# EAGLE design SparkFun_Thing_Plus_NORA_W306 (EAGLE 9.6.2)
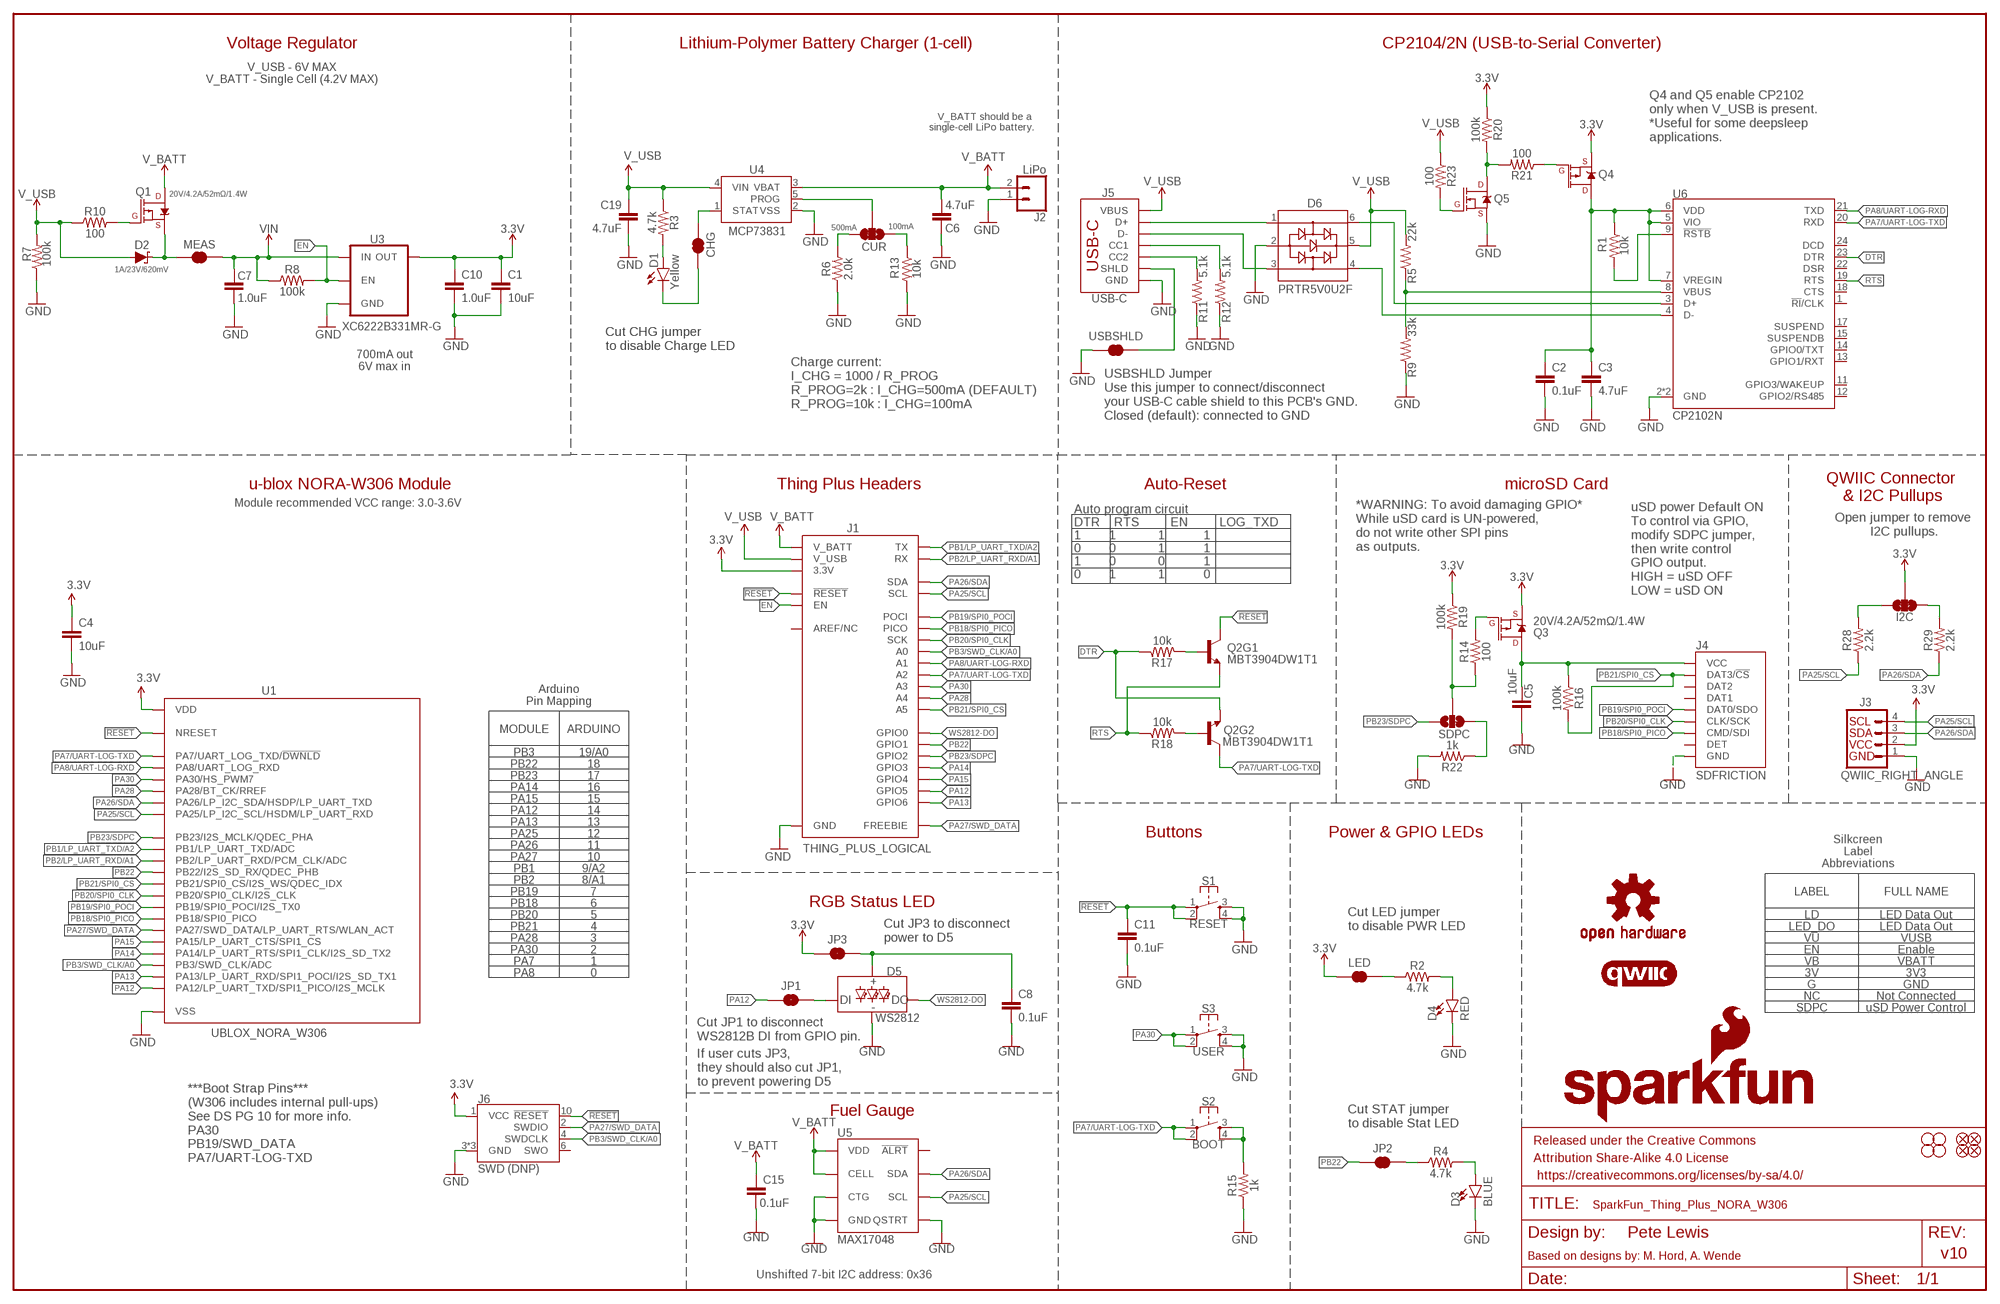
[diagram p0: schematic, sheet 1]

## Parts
C1  10uF  10UF-0402T-6.3V-20%  [0402-TIGHT]
C2  0.1uF  0.1UF-0402T-16V-10%  [0402-TIGHT]
C3  4.7uF  4.7UF-0603-35V-(20%)  [0603]
C4  10uF  10UF-0402T-6.3V-20%  [0402-TIGHT]
C5  10uF  10UF-0402T-6.3V-20%  [0402-TIGHT]
C6  4.7uF  4.7UF-0603-35V-(20%)  [0603]
C7  1.0uF  1.0UF-0402T-16V-10%  [0402-TIGHT]
C8  0.1uF  0.1UF-0402T-16V-10%  [0402-TIGHT]
C10  1.0uF  1.0UF-0402T-16V-10%  [0402-TIGHT]
C11  0.1uF  0.1UF-0402T-16V-10%  [0402-TIGHT]
C15  0.1uF  0.1UF-0402T-16V-10%  [0402-TIGHT]
C19  4.7uF  4.7UF-0603-35V-(20%)  [0603]
CHG  JUMPER-SMT_2_NC_TRACE_SILK  [SMT-JUMPER_2_NC_TRACE_SILK]
CUR  JUMPER-SMT_3_1-NC_TRACE_SILK  [SMT-JUMPER_3_1-NC_TRACE_SILK]
D1  Yellow  LED-YELLOW0603  [LED-0603]
D2  1A/23V/620mV  DIODE-SCHOTTKY-BAT20J  [SOD-323]
D3  BLUE  LED-BLUE0603  [LED-0603]
D4  RED  LED-RED_0603-KB  [LED-0603]
D5  WS2812  WS2812_2020  [WS2812-2020]
D6  PRTR5V0U2F  [SOT886]
FD1  FIDUCIALUFIDUCIAL  [FIDUCIAL-MICRO]
FD2  FIDUCIALUFIDUCIAL  [FIDUCIAL-MICRO]
FD3  FIDUCIALUFIDUCIAL  [FIDUCIAL-MICRO]
FD4  FIDUCIALUFIDUCIAL  [FIDUCIAL-MICRO]
FRAME1  FRAME-LEDGER  [CREATIVE_COMMONS]
H1  STAND-OFF  [STAND-OFF]
H2  STAND-OFF  [STAND-OFF]
H3  STAND-OFF  [STAND-OFF]
H4  STAND-OFF  [STAND-OFF]
I2C  JUMPER-SMT_3_2-NC_TRACE_SILK  [SMT-JUMPER_3_2-NC_TRACE_SILK]
J1  THING_PLUS_LOGICAL  [THING_PLUS]
J2  LiPo  CONN_02-JST-2MM-SMT  [JST-2-SMD]
J3  QWIIC_RIGHT_ANGLE  QWIIC_CONNECTORJS-1MM  [JST04_1MM_RA]
J4  SDFRICTION  MICRO-SDFRICTION  [MICROSD_TINY]
J5  USB-C  USB_C_4-LAYER-ISOLATED  [USB-C-16P-4LAYER-ISOLATED]
J6  SWD (DNP)  CORTEX_JTAG_DEBUG_MINIMUM_SMD_UNSHROUDED_DNP_NO_PASTE  [2X5-SMD-UNSHROUDED_DNP_NO_PASTE]
JP1  JUMPER-SMT_2_NC_TRACE_SILK  [SMT-JUMPER_2_NC_TRACE_SILK]
JP2  JUMPER-SMT_2_NC_TRACE_SILK  [SMT-JUMPER_2_NC_TRACE_SILK]
JP3  JUMPER-SMT_2_NC_TRACE_SILK  [SMT-JUMPER_2_NC_TRACE_SILK]
LED  JUMPER-SMT_2_NC_TRACE_SILK  [SMT-JUMPER_2_NC_TRACE_SILK]
LOGO2  OSHW-LOGOM  [OSHW-LOGO-M]
LOGO3  SFE_LOGO_NAME_FLAME.1_INCH  [SFE_LOGO_NAME_FLAME_.1]
LOGO6  QWIIC_LOGO_4MM  [QWIIC_4MM]
MEAS  JUMPER-COMBO_2_NC_TRACE  [COMBO-JUMPER_2_NC_TRACE]
Q1  20V/4.2A/52mΩ/1.4W  MOSFET_PCH-DMG2305UX-7  [SOT23-3]
Q2  MBT3904DW1T1  TRANS_NPN_DUAL-MBT3904DW1T1  [SC70-6]
Q3  20V/4.2A/52mΩ/1.4W  MOSFET_PCH-DMG2305UX-7  [SOT23-3]
Q4  20V/4.2A/52mΩ/1.4W  MOSFET_PCH-DMG2305UX-7  [SOT23-3]
Q5  20V/0.2A/8MHz/1.2Ω/1Vth  MOSFET-NCH-RE1C002UNTCL  [SOT-416FL]
R1  10k  10KOHM-0402T-1/16W-1%  [0402-TIGHT]
R2  4.7k  4.7KOHM-0402T-1/16W-1%  [0402-TIGHT]
R3  4.7k  4.7KOHM-0402T-1/16W-1%  [0402-TIGHT]
R4  4.7k  4.7KOHM-0402T-1/16W-1%  [0402-TIGHT]
R5  22k  22KOHM-0402_TIGHT-1/10W-1%  [0402-TIGHT]
R6  2.0k  2.0KOHM-0603-1/10W-5%  [0603]
R7  100k  100KOHM-0402T-1/16W-1%  [0402-TIGHT]
R8  100k  100KOHM-0402T-1/16W-1%  [0402-TIGHT]
R9  33k  33KOHM-0402T-1/16W-1%  [0402-TIGHT]
R10  100  100OHM-0402-TIGHT-1/16W-1%  [0402-TIGHT]
R11  5.1k  5.1KOHM-0402T-1/16W-1%  [0402-TIGHT]
R12  5.1k  5.1KOHM-0402T-1/16W-1%  [0402-TIGHT]
R13  10k  10KOHM-0402T-1/16W-1%  [0402-TIGHT]
R14  100  100OHM-0402-TIGHT-1/16W-1%  [0402-TIGHT]
R15  1k  1KOHM-0402T-1/16W-1%  [0402-TIGHT]
R16  100k  100KOHM-0402T-1/16W-1%  [0402-TIGHT]
R17  10k  10KOHM-0402T-1/16W-1%  [0402-TIGHT]
R18  10k  10KOHM-0402T-1/16W-1%  [0402-TIGHT]
R19  100k  100KOHM-0402T-1/16W-1%  [0402-TIGHT]
R20  100k  100KOHM-0402T-1/16W-1%  [0402-TIGHT]
R21  100  100OHM-0402-TIGHT-1/16W-1%  [0402-TIGHT]
R22  1k  1KOHM-0402T-1/16W-1%  [0402-TIGHT]
R23  100  100OHM-0402-TIGHT-1/16W-1%  [0402-TIGHT]
R28  2.2k  2.2KOHM-0402T-1/16W-1%  [0402-TIGHT]
R29  2.2k  2.2KOHM-0402T-1/16W-1%  [0402-TIGHT]
S1  RESET  MOMENTARY-SWITCH-SPST-2-SMD-4.6X2.8MM  [TACTILE_SWITCH_SMD_4.6X2.8MM]
S2  BOOT  MOMENTARY-SWITCH-SPST-2-SMD-4.6X2.8MM  [TACTILE_SWITCH_SMD_4.6X2.8MM]
S3  USER  MOMENTARY-SWITCH-SPST-2-SMD-4.6X2.8MM  [TACTILE_SWITCH_SMD_4.6X2.8MM]
SDPC  JUMPER-SMT_3_1-NC_TRACE_SILK  [SMT-JUMPER_3_1-NC_TRACE_SILK]
U1  UBLOX_NORA_W306  [UBLOX-NORA-W3]
U3  XC6222B331MR-G  [SOT23-5]
U4  MCP73831  [SOT23-5]
U5  MAX17048  MAX17048DFN8  [DFN-8]
U6  CP2102N  [QFN24]
USBSHLD  JUMPER-SMT_2_NC_TRACE_SILK  [SMT-JUMPER_2_NC_TRACE_SILK]

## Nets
3.3V: C1.1 C4.1 C10.1 I2C.2 J1.27(3.3V) J3.2 J6.1(VCC) JP3.1 LED.1 Q3.2(S) Q4.2(S) R19.1 R20.1 U1.A7(VDD) U1.A8(VDD) U1.B7(VDD) U3.5(OUT)
!RESET!: C11.1 J1.28(!RESET) J6.10(!RESET) Q2.3(C) S1.1 S1.2 U1.J3(NRESET)
CC1: J5.A5(CC1) R12.2
CC2: J5.B5(CC2) R11.2
CHG: CHG.2 U4.1(STAT)
DTR: Q2.1(E) R17.1 U6.23(DTR)
EN: J1.11(EN) R8.2 U3.3(EN)
GND: C1.2 C2.2 C3.2 C4.2 C5.2 C6.2 C7.2 C8.2 C10.2 C11.2 C15.2 C19.2 D3.C D4.C D5.GND D6.2 J1.25(GND) J2.1 J3.1 J4.6(GND) J4.GND1(GND) J4.GND2(GND) J4.GND3(GND) J4.GND4(GND) J4.GND5(GND) J4.GND6(GND) J5.GND J5.GND2(GND) J6.3(GND) J6.5(GND) J6.9(GND) Q5.2(S) R6.1 R7.1 R9.1 R11.1 R12.1 R13.2 R15.1 R22.2 S1.3 S1.4 S3.3 S3.4 U1.A1(VSS) U1.A9(VSS) U1.B2(VSS) U1.B8(VSS) U1.E4(VSS) U1.E5(VSS) U1.F4(VSS) U1.F5(VSS) U1.K2(VSS) U1.K3(VSS) U1.K5(VSS) U1.K7(VSS) U1.K8(VSS) U1.L1(VSS) U1.L9(VSS) U1.M1(VSS) U1.M2(VSS) U1.M8(VSS) U1.M9(VSS) U3.2(GND) U4.2(VSS) U5.1(CTG) U5.4(GND) U5.6(QSTRT) U5.9(GND) U6.2(GND) U6.PAD(GND) USBSHLD.1
N$1: R1.2 U6.9(!RSTB)
N$2: D3.A R4.2
N$3: Q2.5(B) R17.2
N$4: R5.1 R9.2 U6.8(VBUS)
N$5: Q2.2(B) R18.2
N$6: CHG.1 D1.C
N$7: Q1.1(G) R10.2
N$8: R15.2 S2.3 S2.4
N$9: CUR.2 U4.5(PROG)
N$10: D5.DI JP1.2
N$11: CUR.1 R13.1
N$12: LED.2 R2.1
N$13: CUR.3 R6.2
N$14: D4.A R2.2
N$15: D6.6 U6.3(D+)
N$16: D6.1 J5.A6(D+) J5.B6(D+)
N$17: D1.A R3.2
N$18: D6.4 U6.4(D-)
N$19: D6.3 J5.A7(D-) J5.B7(D-)
N$20: I2C.3 R28.2
N$21: I2C.1 R29.2
N$22: JP2.2 R4.1
N$23: D2.C MEAS.1 MEAS.3 Q1.2(S)
N$24: Q3.1(G) R14.2
N$25: C5.1 J4.4(VCC) Q3.3(D) R16.1
N$26: R14.1 R19.2 SDPC.2
N$27: Q5.3(D) R20.2 R21.2
N$28: C8.1 D5.VCC JP3.2
N$29: C2.1 C3.1 Q4.3(D) R1.1 U6.5(VIO) U6.6(VDD) U6.7(VREGIN)
N$30: Q4.1(G) R21.1
N$31: Q5.1(G) R23.2
N$32: R22.1 SDPC.3
PA7/UART-LOG-TXD: J1.22(A2) Q2.6(C) S2.1 S2.2 U1.A5(PA7/UART_LOG_TXD/!DWNLD!) U6.20(RXD)
PA8/UART-LOG-RXD: J1.23(A1) U1.A6(PA8/UART_LOG_RXD) U6.21(TXD)
PA12: J1.4(GPIO5) JP1.1 U1.J9(PA12/LP_UART_TXD/SPI1_PICO/I2S_MCLK)
PA13: J1.3(GPIO6) U1.J8(PA13/LP_UART_RXD/SPI1_POCI/I2S_SD_TX1)
PA14: J1.6(GPIO3) U1.H9(PA14/LP_UART_RTS/SPI1_CLK/I2S_SD_TX2)
PA15: J1.5(GPIO4) U1.H8(PA15/LP_UART_CTS/SPI1_CS)
PA25/SCL: J1.2(SCL) J3.4 R28.1 U1.C2(PA25/LP_I2C_SCL/HSDM/LP_UART_RXD) U5.7(SCL)
PA26/SDA: J1.1(SDA) J3.3 R29.1 U1.C1(PA26/LP_I2C_SDA/HSDP/LP_UART_TXD) U5.8(SDA)
PA27/SWD_DATA: J1.13(FREEBIE) J6.2(SWDIO) U1.H2(PA27/SWD_DATA/LP_UART_RTS/WLAN_ACT)
PA28: J1.20(A4) U1.B3(PA28/BT_CK/RREF)
PA30: J1.21(A3) S3.1 S3.2 U1.B1(PA30/HS_PWM7)
PB1/LP_UART_TXD/A2: J1.14(TX) U1.D8(PB1/LP_UART_TXD/ADC)
PB2/LP_UART_RXD/A1: J1.15(RX) U1.E8(PB2/LP_UART_RXD/PCM_CLK/ADC)
PB3/SWD_CLK/A0: J1.24(A0) J6.4(SWDCLK) U1.J2(PB3/SWD_CLK/ADC)
PB18/SPI0_PICO: J1.17(PICO) J4.3(CMD/SDI) U1.G9(PB18/SPI0_PICO)
PB19/SPI0_POCI: J1.16(POCI) J4.7(DAT0/SDO) U1.G8(PB19/SPI0_POCI/I2S_TX0)
PB20/SPI0_CLK: J1.18(SCK) J4.5(CLK/SCK) U1.F9(PB20/SPI0_CLK/I2S_CLK)
PB21/SPI0_CS: J1.19(A5) J4.2(DAT3/!CS!) R16.2 U1.F8(PB21/SPI0_CS/I2S_WS/QDEC_IDX)
PB22: J1.8(GPIO1) JP2.1 U1.E9(PB22/I2S_SD_RX/QDEC_PHB)
PB23/SDPC: J1.7(GPIO2) SDPC.1 U1.C8(PB23/I2S_MCLK/QDEC_PHA)
RTS: Q2.4(E) R18.1 U6.19(RTS)
USB_SHLD: J5.SHLD1(SHLD) J5.SHLD2(SHLD) J5.SHLD3(SHLD) J5.SHLD4(SHLD) J5.SHLD5(SHLD) J5.SHLD6(SHLD) J5.SHLD7(SHLD) J5.SHLD8(SHLD) USBSHLD.2
V_BATT: C6.1 C15.1 J1.12(V_BATT) J2.2 Q1.3(D) U4.3(VBAT) U5.2(CELL) U5.3(VDD)
V_USB: C19.1 D2.A D6.5 J1.10(V_USB) J5.VBUS1(VBUS) J5.VBUS2(VBUS) R3.1 R5.2 R7.2 R10.1 R23.1 U4.4(VIN)
VIN: C7.1 MEAS.2 MEAS.4 R8.1 U3.1(IN)
WS2812-DO: D5.DO J1.9(GPIO0)
Unconnected: J1.26(AREF/NC) J4.1(DAT2) J4.8(DAT1) J4.9(DET) J6.6(SWO) U5.5(!ALRT) U6.1(!RI!/CLK) U6.11(GPIO3/WAKEUP) U6.12(GPIO2/RS485) U6.13(GPIO1/RXT) U6.14(GPIO0/TXT) U6.15(SUSPENDB) U6.17(SUSPEND) U6.18(CTS) U6.22(DSR) U6.24(DCD)

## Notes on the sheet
- Voltage Regulator | Lithium-Polymer Battery Charger (1-cell) | CP2104/2N (USB-to-Serial Converter)
- V_USB - 6V MAX
  V_BATT - Single Cell (4.2V MAX)
- V_BATT should be a 
  single-cell LiPo battery.
- Q4 and Q5 enable CP2102
  only when V_USB is present.
  *Useful for some deepsleep 
  applications.
- 500mA | 100mA
- 700mA out
  6V max in
- Cut CHG jumper 
  to disable Charge LED
- Charge current:
  I_CHG = 1000 / R_PROG
  R_PROG=2k : I_CHG=500mA (DEFAULT)
  R_PROG=10k : I_CHG=100mA
- USBSHLD Jumper
  Use this jumper to connect/disconnect
  your USB-C cable shield to this PCB's GND.
  Closed (default): connected to GND
- u-blox NORA-W306 Module | Thing Plus Headers | Auto-Reset | microSD Card
- QWIIC Connector 
  & I2C Pullups
- Module recommended VCC range: 3.0-3.6V
- *WARNING: To avoid damaging GPIO*
  While uSD card is UN-powered,
  do not write other SPI pins
  as outputs.
- Open jumper to remove 
  I2C pullups.
- uSD power Default ON
  To control via GPIO, 
  modify SDPC jumper,
  then write control 
  GPIO output.
  HIGH = uSD OFF
  LOW = uSD ON
- Auto program circuit
  DTR    RTS         EN         LOG_TXD
  1        1            1           1
  0        0            1           1
  1        0            0           1
  0        1            1           0
- Arduino
  Pin Mapping
- MODULE | ARDUINO
- PB3 | 19/A0
- PB22 | 18
- PB23 | 17
- PA14 | 16
- PA15 | 15
- PA12 | 14
- PA13 | 13
- PA25 | 12 | Buttons | Power & GPIO LEDs
- PA26 | 11
- PA27 | 10
- Silkcreen
  Label
  Abbreviations
- PB1 | 9/A2
- PB2 | 8/A1
- PB19 | 7 | LABEL | FULL NAME
- PB18 | 6 | RGB Status LED
- PB20 | 5 | LD | LED Data Out
- PB21 | 4
- Cut LED jumper 
  to disable PWR LED
- LED_DO | LED Data Out
- PA28 | 3
- Cut JP3 to disconnect
  power to D5
- VU | VUSB
- PA30 | 2 | EN | Enable
- PA7 | 1 | VB | VBATT
- PA8 | 0 | 3V | 3V3
- G | GND
- NC | Not Connected
- SDPC | uSD Power Control
- Cut JP1 to disconnect
  WS2812B DI from GPIO pin.
- If user cuts JP3,
  they should also cut JP1,
  to prevent powering D5
- Fuel Gauge
- Cut STAT jumper 
  to disable Stat LED
- ***Boot Strap Pins***
  (W306 includes internal pull-ups)
  See DS PG 10 for more info.
  PA30
  PB19/SWD_DATA
  PA7/UART-LOG-TXD
- Pete Lewis
- v10
- Based on designs by: M. Hord, A. Wende
- Unshifted 7-bit I2C address: 0x36

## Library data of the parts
C1 C4 C5 = SparkFun-Capacitors:10UF: 10.0µF ceramic capacitors; PROD_ID: CAP-14848
C2 C8 C11 C15 = SparkFun-Capacitors:0.1UF: 0.1µF ceramic capacitors; PROD_ID: CAP-12416
C3 C6 C19 = SparkFun-Capacitors:4.7UF: 4.7µF ceramic capacitors; PROD_ID: CAP-14106
C7 C10 = SparkFun-Capacitors:1.0UF: 1µF ceramic capacitors; PROD_ID: CAP-12417
CHG JP1-JP3 LED USBSHLD = SparkFun-Jumpers:JUMPER-SMT_2_NC_TRACE: Normally closed trace jumper
CUR SDPC = SparkFun-Jumpers:JUMPER-SMT_3_1-NC_TRACE: Normally closed trace jumper (1 of 2 connections) This jumper has a trace between two pads so it's normally closed (NC). The other connection is normally open (NO). Use a razor knife to open the connection. For best results follow the IPC guidelines for cutting traces: Cutout at least 0.063 mm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
D1 = SparkFun-LED:LED-YELLOW: Yellow SMD LED; PROD_ID: DIO-09003
D2 = SparkFun-DiscreteSemi:DIODE-SCHOTTKY: Schottky diode; PROD_ID: DIO-11623
D3 = SparkFun-LED:LED-BLUE: Blue SMD LED; PROD_ID: DIO-08575
D4 = SparkFun-LED:LED-RED: Red SMD LED; PROD_ID: DIO-17976
D5 = SparkFun-LED:WS2812: Addressable RGB LED - 1 Wire Common names: WS2812, SK6812, Neopixel, APA-106, etc. SMD LED with built-in controller IC. Color: Red/Green/Blue SparkFun Products: LED-SMD RGB (WS2812) LED - RGB Addressable, PTH, 5mm Diffused (5 Pack) LED - RGB Addressable, PTH, 5mm Clear (5 Pack) Blynk Board -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; PROD_ID: DIO-15591
D6 = SparkFun-IC-Power:PRTR5V0U2: A small ESD protection device. Most commonly used on USB D+/D- signals to protect large, expensive, or especially sensitive USB enabled devices.; PROD_ID: DIO-14084
FD1-FD4 = SparkFun-Aesthetics:FIDUCIAL: Fiducial Alignment Points
FRAME1 = SparkFun-Aesthetics:FRAME-LEDGER: Schematic Frame - Ledger
H1-H4 = SparkFun-Hardware:STAND-OFF: Stand Off
I2C = SparkFun-Jumpers:JUMPER-SMT_3_2-NC_TRACE: Normally closed trace jumper (2 of 2 connections) This jumper has a trace between all three pads so they are normally closed (NC). Use a razor knife to open the connection(s). For best results follow the IPC guidelines for cutting traces: Cutout at least 0.063 mm (0.005 in). Remove all loose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
J1 = SparkFun-Boards:THING_PLUS_LOGICAL
J2 = SparkFun-Connectors:CONN_02: Multi connection point. Often used as Generic Header-pin footprint for 0.1 inch spaced/style header connections; PROD_ID: CONN-11443
J3 = SparkFun-Connectors:QWIIC_CONNECTOR: SparkFun I2C Standard Qwiic Connector An SMD 1mm pitch JST connector makes it easy and quick (get it? Qwiic?) to connect I2C devices to each other. The Qwiic system enables fast and solderless connection between popular platforms and various sensors and actuators. We carry 200mm, 100mm, 50mm, and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; PROD_ID: CONN-13694
J4 = SparkFun-Connectors:MICRO-SD: microSD Socket for Transflash Various sockets for µSD. tDoc lines correctly indicate media card edge positions when inserting (unlocked, locked, depressed). NOTE: CD1 and CD2 are connected internally, and the default detect state of the socket is detect pin to ground. SparkFun Products: WAV Trigger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; PROD_ID: CONN-13500
J5 = SparkFun-Connectors:USB_C: USB Type C 16Pin Connector Super Speed pins not available on the 16-pin purely SMD connector so this part is best for USB 2.0 implementations. D1 and D2 are tied together enabling D+/- no matter which way the cable is plugged into the connector. The two channel configuration pins (CC1/2) are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; PROD_ID: CONN-14122; VALUE: USB Female Type C Connector
J6 = SparkFun-Connectors:CORTEX_JTAG_DEBUG_MINIMUM: Cortex Debug Connector - 10 pin Supports JTAG debug, Serial Wire debug, and Serial Wire Viewer. PTH and SMD connector options available. General Connector Information Products: PTH Connector -via Digi-Key SparkFun PSoc SparkFun T
LOGO2 = SparkFun-Aesthetics:OSHW-LOGO: Open-Source Hardware (OSHW) Logo
LOGO3 = SparkFun-Aesthetics:SFE_LOGO_NAME_FLAME: SparkFun Font Logo w/ Flame
LOGO6 = SparkFun-Aesthetics:QWIIC_LOGO: Qwiic Logos for placement on schematic and PCB. The 5.5mm silk logo is best for placing next to Qwiic connector.
MEAS = SparkFun-Jumpers:JUMPER-COMBO_2_NC_TRACE
Q1 Q3 Q4 = SparkFun-DiscreteSemi:MOSFET_PCH: P-channel MOSFETs Voltage controlled devices that allow control of high current outputs. SparkFun Products: SparkFun ESP32 Thing SparkFun ESP8266 Thing SparkFun Pi Servo HAT V2 DMG2305UX-7 (20V/4.2A/SOT23-3); PROD_ID: TRANS-14388
Q2 = SparkFun-DiscreteSemi:TRANS_NPN_DUAL: Dual NPN Transistors in Single Package The MBT3904W1 puts two general purpose 3904 NPN transistors in a single package. Datasheet SparkFun Products: SparkFun ESP32 Thing; PROD_ID: TRANS-13337
Q5 = SparkFun-DiscreteSemi:MOSFET-NCH: N-channel MOSFETs Voltage controlled devices that allow control of high current outputs. SparkFun Products: SparkFun OpenScale SparkFun Digital Sandbox SparkFun Monster Moto Shield SparkFun MOSFET Power Controller; PROD_ID: TRANS-14399
R1 R13 R17 R18 = SparkFun-Resistors:10KOHM: 10kΩ resistor; PROD_ID: RES-14241
R2-R4 = SparkFun-Resistors:4.7KOHM: 4.7kΩ resistor; PROD_ID: RES-15343
R5 = SparkFun-Resistors:22KOHM: 22kΩ resistor; PROD_ID: RES-14281
R6 = SparkFun-Resistors:2.0KOHM: 2kΩ resistor; PROD_ID: RES-08296
R7 R8 R16 R19 R20 = SparkFun-Resistors:100KOHM: 100kΩ resistor; PROD_ID: RES-13495
R9 = SparkFun-Resistors:33KOHM: 33kΩ resistor; PROD_ID: RES-15128
R10 R14 R21 R23 = SparkFun-Resistors:100OHM: 100Ω resistor; PROD_ID: RES-14962
R11 R12 = SparkFun-Resistors:5.1KOHM; PROD_ID: RES-14340
R15 R22 = SparkFun-Resistors:1KOHM: 1kΩ resistor; PROD_ID: RES-14342
R28 R29 = SparkFun-Resistors:2.2KOHM: 2.2kΩ resistor; PROD_ID: RES-14341
S1-S3 = SparkFun-Switches:MOMENTARY-SWITCH-SPST-2: Momentary Switch (Pushbutton) - SPST - Two Circuits Normally-open (NO) SPST momentary switches (buttons, pushbuttons). Schematic symbol includes two switch circuits. Variants SMD-4.6MMX2.8MM - 4.60mm x 2.80mm Tactile Momentary Button Switch - Used on SparkFun Pro Micro - RP2040 SMD-5.2MM - Mini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; PROD_ID: SWCH-15606
U1 = nora-w306:UBLOX_NORA_W306; PROD_ID: IC-17585
U3 = SparkFun-IC-Power:XC6222; IOUT: 700mA; PROD_ID: VREG-16775; VOUT: 3.3V
U4 = SparkFun-IC-Power:MCP73831: MCP73831T Li-Ion, Li-Pol Controller Miniature single cell, fully integrated Li-Ion, Li-polymer charge management controller Datasheet SparkFun Products: SparkFun ESP32 Thing SparkFun 9DoF Razor IMU M0; PROD_ID: IC-09995
U5 = SparkFun-IC-Power:MAX17048: Micropower 1-Cell Li+ ModelGauge SparkFun Products Qduino Mini (DEV-13614); PROD_ID: IC-12551
U6 = SparkFun-IC-Comms:CP2102N; PROD_ID: IC-14020

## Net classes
0 default: width 0 mm, drill 0 mm
1 POWER: width 0.559 mm, drill 0.305 mm

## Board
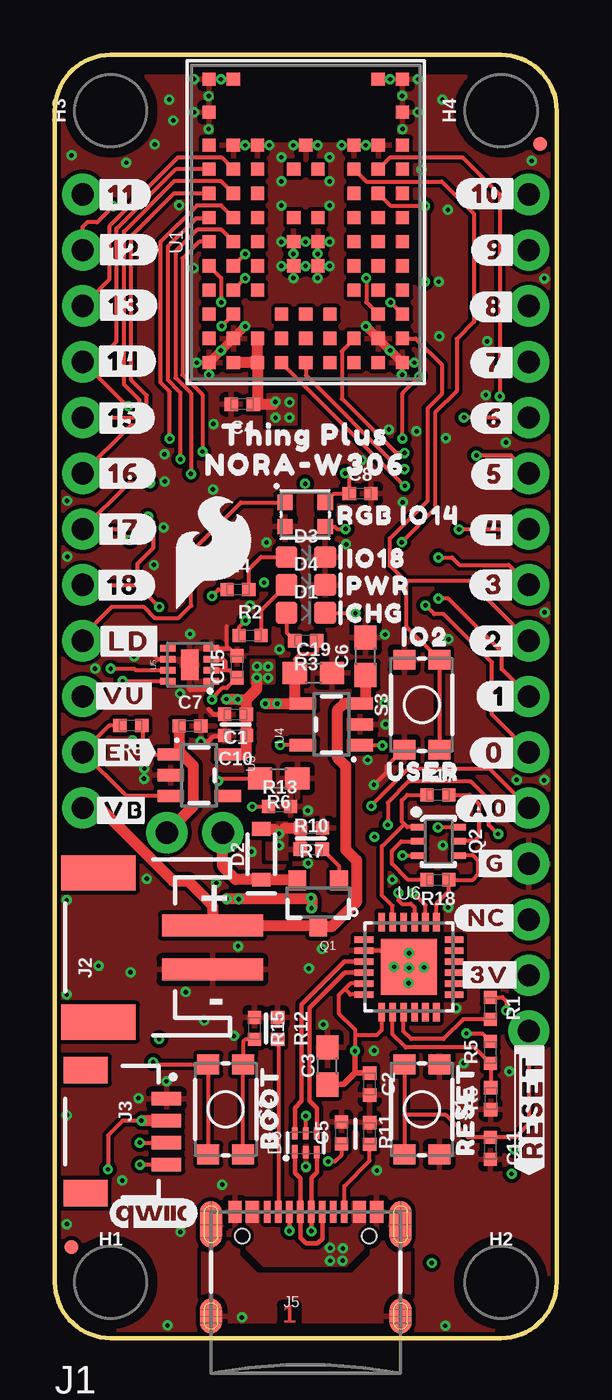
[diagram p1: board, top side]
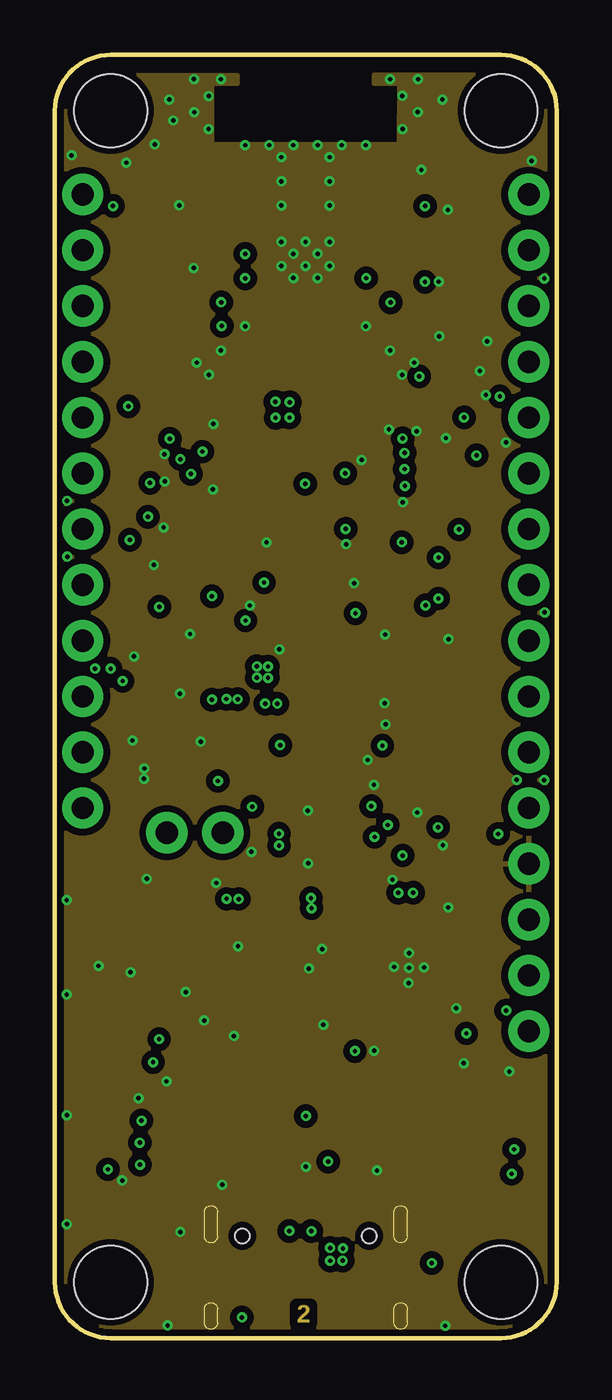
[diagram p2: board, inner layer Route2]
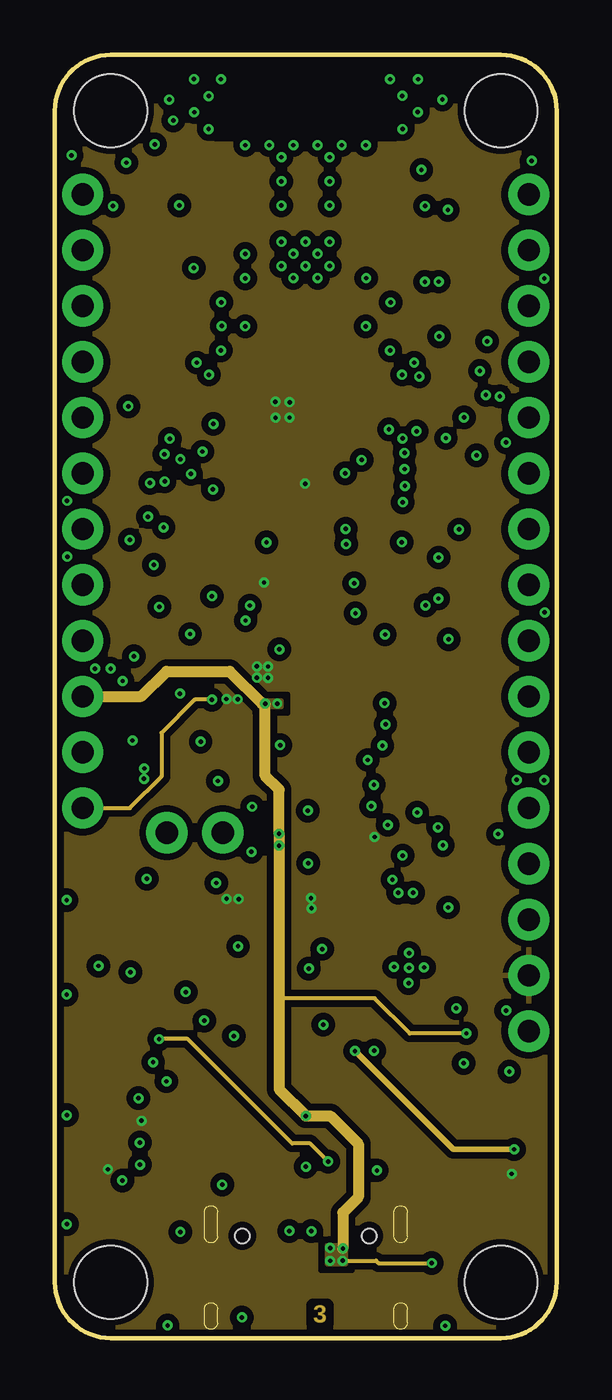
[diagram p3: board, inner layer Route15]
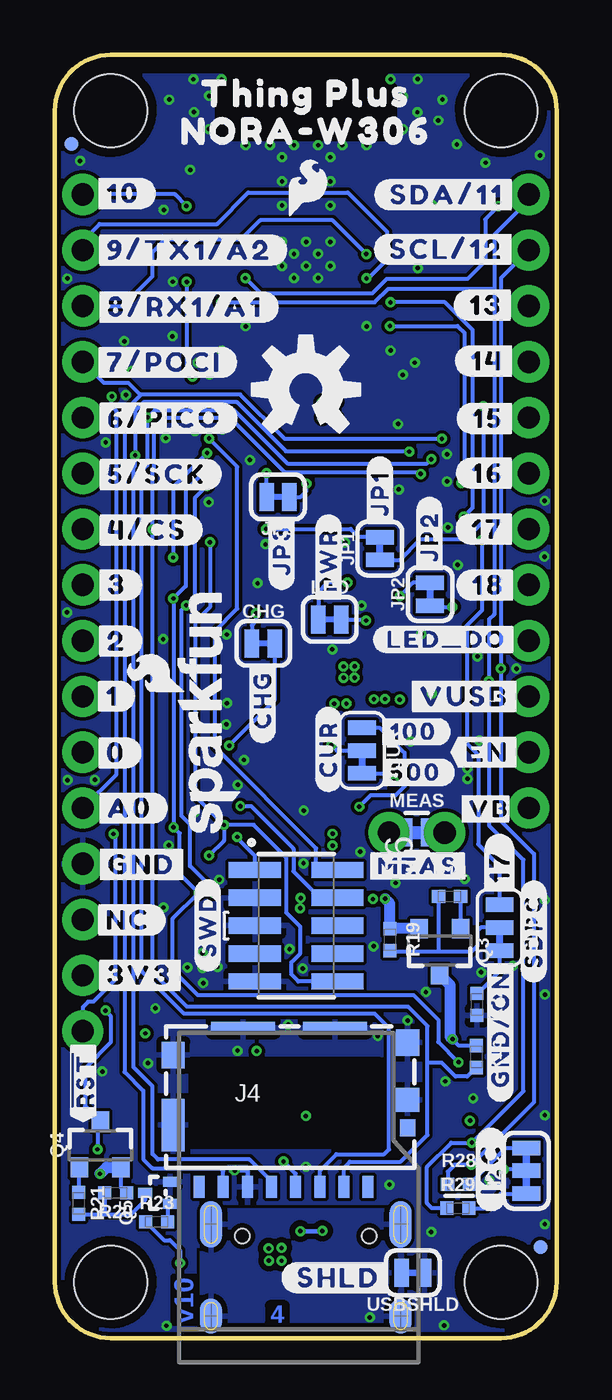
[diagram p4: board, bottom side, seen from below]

Size 22.86 x 58.42 mm. Coordinates in mm from the lower left corner, seen from the top.
Outline: 22.86,2.54 22.86,55.88 arc90 20.32,58.42 2.54,58.42 arc90 0,55.88 0,2.54 arc90 2.54,0 20.32,0 arc90 22.86,2.54
Copper layers (1*2*15*16): Top 0.035559375mm / dielectric 0.47751875mm / Route2 0.035559375mm / dielectric 0.47751875mm / Route15 0.035559375mm / dielectric 0.47751875mm / Bottom 0.035559375mm
Design rules "SparkFun-4-Layer-Minimum-JLCPCB": minimum track width 5mil, minimum drill 0.2mm, track to track 5mil, track to pad 5mil, pad to pad 5mil, via to via 5mil, smd to smd 5mil, copper to edge 7mil, drill to drill 7mil, minimum pad ring 5mil, minimum via ring 5mil, stop-mask expansion 2.5mil, vias tented up to drill 25mil, thermal gap 10mil
tRestrict: area 17.6,16.8 to 17.6,17; area 16.1,18.3 to 16.2,18.4; area 14.7,16.8 to 14.7,17; area 16.1,15.4 to 16.2,15.5

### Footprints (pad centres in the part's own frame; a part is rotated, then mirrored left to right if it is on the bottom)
0402-TIGHT = smd 0.6 x 0.6: 1 -0.5,0; 2 0.5,0
0603 = smd 1.1 x 1: 1 -0.85,0; 2 0.85,0
SMT-JUMPER_2_NC_TRACE_SILK = smd 0.66 x 1.27: 1 -0.521,0; 2 0.521,0
SMT-JUMPER_3_1-NC_TRACE_SILK = smd 0.66 x 1.27: 1 -1.041,0; 2 0,0; 3 1.041,0
LED-0603 = smd 1 x 1: A -0.877,0; C 0.877,0
SOD-323 = smd 0.63 x 0.83: A 1.15,0; C -1.15,0
WS2812-2020 = smd 0.7 x 0.7: DI -0.915,0.55; DO 0.915,-0.55; GND 0.915,0.55; VCC -0.915,-0.55
SOT886 = smd 0.61 x 0.25: 1 -0.405,0.5 | smd 0.56 x 0.25: 2 -0.43,0; 3 -0.43,-0.5; 4 0.43,-0.5; 5 0.43,0; 6 0.43,0.5
FIDUCIAL-MICRO = smd 0.635 x 0.635: 1 0,0
STAND-OFF = hole 3.302: 0,0
SMT-JUMPER_3_2-NC_TRACE_SILK = smd 0.66 x 1.27: 1 -1.041,0; 2 0,0; 3 1.041,0
THING_PLUS = drill 1.016 pad 1.88: 1 1.27,52.07; 2 1.27,49.53; 3 1.27,46.99; 4 1.27,44.45; 5 1.27,41.91; 6 1.27,39.37; 7 1.27,36.83; 8 1.27,34.29; 9 1.27,31.75; 10 1.27,29.21; 11 1.27,26.67; 12 1.27,24.13; 13 21.59,52.07; 14 21.59,49.53; 15 21.59,46.99; 16 21.59,44.45; 17 21.59,41.91; 18 21.59,39.37; 19 21.59,36.83; 20 21.59,34.29; 21 21.59,31.75; 22 21.59,29.21; 23 21.59,26.67; 24 21.59,24.13; 25 21.59,21.59; 26 21.59,19.05; 27 21.59,16.51; 28 21.59,13.97
JST-2-SMD = smd 1 x 4.6: 1 -1,-3.7; 2 1,-3.7 | smd 1.6 x 3.4: NC1 -3.4,1.5; NC2 3.4,1.5
JST04_1MM_RA = smd 0.6 x 1.35: 1 -1.5,0; 2 -0.5,0; 3 0.5,0; 4 1.5,0 | smd 1.2 x 2: NC1 2.8,-3.675; NC2 -2.8,-3.675
MICROSD_TINY = smd 0.5 x 1: 1 3.55,-3.85; 2 2.45,-3.85; 3 1.35,-3.85; 4 0.25,-3.85; 5 -0.85,-3.85; 6 -1.95,-3.85; 7 -3.05,-3.85; 8 -4.15,-3.85 | smd 0.72 x 0.78: 9 5.35,-1.17 | smd 1.05 x 1.08: GND1 5.35,0.1 | smd 1.05 x 1.2: GND2 5.35,2.71; GND3 -5.325,2.14 | smd 1.05 x 2.39: GND4 -5.325,-1.045 | smd 2.91 x 0.55: GND5 -2.145,3.385; GND6 2.045,3.385
USB-C-16P-4LAYER-ISOLATED = smd 0.3 x 1: A5 -1.25,-0.34; A6 -0.25,-0.34; A7 0.25,-0.34; A8 1.25,-0.34; B5 1.75,-0.34; B6 0.75,-0.34; B7 -0.75,-0.34; B8 -1.75,-0.34 | smd 0.6 x 1: GND -3.225,-0.34; GND2 3.225,-0.34; VBUS1 -2.45,-0.34; VBUS2 2.45,-0.34 | smd 1 x 2.1: SHLD1 -4.32,-0.915; SHLD2 4.32,-0.915 | smd 1 x 2.1 bottom: SHLD3 -4.32,-0.915; SHLD4 4.32,-0.915 | smd 1 x 1.6: SHLD5 -4.32,-5.095; SHLD8 4.32,-5.095 | smd 1 x 1.6 bottom: SHLD6 -4.32,-5.095; SHLD7 4.32,-5.095 | hole 0.65: -2.89,-1.445; 2.89,-1.445
2X5-SMD-UNSHROUDED_DNP_NO_PASTE = smd 0.74 x 2.38: 1 -2.54,-1.88; 2 -2.54,1.88; 3 -1.27,-1.88; 4 -1.27,1.88; 5 0,-1.88; 6 0,1.88; 7 1.27,-1.88; 8 1.27,1.88; 9 2.54,-1.88; 10 2.54,1.88
COMBO-JUMPER_2_NC_TRACE = smd 0.635 x 1.27: 1 -0.508,0; 2 0.508,0 | drill 1.016 pad 1.88: 3 -1.27,0; 4 1.27,0
SOT23-3 = smd 0.8 x 0.9: 1 -0.95,-1; 2 0.95,-1; 3 0,1.1
SC70-6 = smd 0.3 x 0.66: 1 -0.65,-0.92; 2 0,-0.92; 3 0.65,-0.92; 4 0.65,0.92; 5 0,0.92; 6 -0.65,0.92
SOT-416FL = smd 0.46 x 0.65: 1 -0.5,-1.1; 2 0.5,-1.1; 3 0,0.05
TACTILE_SWITCH_SMD_4.6X2.8MM = smd 0.9 x 1: 1 -2.05,-0.8; 2 2.05,-0.8; 3 2.05,0.8; 4 -2.05,0.8
UBLOX-NORA-W3 = smd 0.6 x 0.6: A1 -5.5,-4.4; A2 -5.5,-3.3; A3 -5.5,-2.2; A4 -5.5,-1.1; A5 -5.5,0; A6 -5.5,1.1; A7 -5.5,2.2; A8 -5.5,3.3; A9 -5.5,4.4; B1 -4.4,-4.4; B2 -4.4,-3.3; B3 -4.4,-2.2; B4 -4.4,-1.1; B5 -4.4,0; B6 -4.4,1.1; B7 -4.4,2.2; B8 -4.4,3.3; B9 -4.4,4.4; C1 -3.3,-4.4; C2 -3.3,-3.3; C4 -3.3,-1.1; C5 -3.3,0; C6 -3.3,1.1; C8 -3.3,3.3; C9 -3.3,4.4; D1 -2.2,-4.4; D2 -2.2,-3.3; D3 -2.2,-2.2; D7 -2.2,2.2; D8 -2.2,3.3; D9 -2.2,4.4; E1 -1.1,-4.4; E2 -1.1,-3.3; E3 -1.1,-2.2; E4 -1.1,-0.55; E5 -1.1,0.55; E7 -1.1,2.2; E8 -1.1,3.3; E9 -1.1,4.4; F1 0,-4.4; F2 0,-3.3; F3 0,-2.2; F4 0,-0.55; F5 0,0.55; F7 0,2.2; F8 0,3.3; F9 0,4.4; G1 1.1,-4.4; G2 1.1,-3.3; G3 1.1,-2.2; G4 1.1,-0.55; G5 1.1,0.55; G7 1.1,2.2; G8 1.1,3.3; G9 1.1,4.4; H1 2.2,-4.4; H2 2.2,-3.3; H3 2.2,-2.2; H7 2.2,2.2; H8 2.2,3.3; H9 2.2,4.4; J1 3.3,-4.4; J2 3.3,-3.3; J3 3.3,-2.2; J4 3.3,-0.55; J5 3.3,0.55; J7 3.3,2.2; J8 3.3,3.3; J9 3.3,4.4; K1 4.4,-4.4; K2 4.4,-3.3; K3 4.4,-2.2; K5 4.4,0; K7 4.4,2.2; K8 4.4,3.3; K9 4.4,4.4; L1 5.9,-4.4; L9 5.9,4.4; M1 7.4,-4.4; M2 7.4,-3.3; M8 7.4,3.3; M9 7.4,4.4
SOT23-5 = smd 0.55 x 1.2: 1 -0.95,-1.3; 2 0,-1.3; 3 0.95,-1.3; 4 0.95,1.3; 5 -0.95,1.3
DFN-8 = smd 0.3 x 0.7: 1 -0.75,-0.99; 2 -0.25,-0.99; 3 0.25,-0.99; 4 0.75,-0.99; 5 0.75,0.99; 6 0.25,0.99; 7 -0.25,0.99; 8 -0.75,0.99 | smd 1.38 x 0.8: 9 0,0
QFN24 = smd 0.85 x 0.3: 1 -2.05,1.25; 2 -2.05,0.75; 3 -2.05,0.25; 4 -2.05,-0.25; 5 -2.05,-0.75; 6 -2.05,-1.25; 13 2.05,-1.25; 14 2.05,-0.75; 15 2.05,-0.25; 16 2.05,0.25; 17 2.05,0.75; 18 2.05,1.25 | smd 0.3 x 0.85: 7 -1.25,-2.05; 8 -0.75,-2.05; 9 -0.25,-2.05; 10 0.25,-2.05; 11 0.75,-2.05; 12 1.25,-2.05; 19 1.25,2.05; 20 0.75,2.05; 21 0.25,2.05; 22 -0.25,2.05; 23 -0.75,2.05; 24 -1.25,2.05 | smd 2.55 x 2.55: PAD 0,0

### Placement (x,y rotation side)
C1  8.22,28.4 180 top
C2  14.34,11.56 270 top
C3  12.41,12.39 90 top
C4  8.53,42.51 180 top
C5  13.05,9.34 90 top
C6  14.15,31.04 90 top
C7  6.15,27.87 0 top
C8  13.9,38.45 0 top
C10  8.23,27.43 180 top
C11  19.83,8.64 270 top
C15  8.3,30.56 90 top
C19  11.78,30.27 0 top
CHG  13.36,31.63 0 bottom
CUR  8.86,26.75 270 bottom
D1  11.43,33.02 0 top
D2  9.4,22.02 90 top
D3  11.43,35.56 0 top
D4  11.43,34.29 0 top
D5  11.4,37.5 180 top
D6  11.43,8.89 90 top
FD1  22.1,54.36 0 top
FD2  22.1,54.36 0 bottom
FD3  0.74,4.14 0 top
FD4  0.74,4.14 0 bottom
FRAME1  not placed on the board
H1  2.54,2.54 0 top
H2  20.32,2.54 0 top
H3  2.54,55.88 90 top
H4  20.32,55.88 90 top
I2C  1.39,7.62 90 bottom
J1  0,0 0 top
J2  3.48,17.78 90 top
J3  5.08,9.4 270 top
J4  12.14,10.74 0 bottom
J5  11.43,6.1 0 top
J6  11.87,18.78 270 bottom
JP1  8.06,35.95 90 bottom
JP2  5.77,33.87 90 bottom
JP3  12.7,38.3 180 bottom
LED  10.34,32.72 0 bottom
LOGO2  11.43,43.18 0 bottom
LOGO3  15.87,28.54 90 bottom
LOGO6  4.5,5.67 0 top
MEAS  6.38,23.01 0 bottom
Q1  11.99,19.84 180 top
Q2  17.47,22.62 270 top
Q3  5.33,17.64 180 bottom
Q4  20.79,8.77 0 bottom
Q5  18.7,6.62 90 bottom
R1  19.83,15.01 270 top
R2  8.89,31.98 0 top
R3  11.43,31.75 180 top
R4  8.34,34.08 0 top
R5  19.83,13.01 90 top
R6  10.19,25.47 180 top
R7  11.69,23.22 180 top
R8  3.46,27.88 180 top
R9  19.85,10.9 90 top
R10  11.68,22.25 0 top
R11  14.34,9.31 270 top
R12  10.15,14.09 270 top
R13  10.24,24.21 0 top
R14  4.88,20.1 0 bottom
R15  9.09,14.1 270 top
R16  3.67,12.81 270 bottom
R17  17.45,24.73 0 top
R18  17.45,20.87 180 top
R19  7.6,18.14 270 bottom
R20  20.09,6.61 180 bottom
R21  21.77,6.14 270 bottom
R22  3.64,15.19 270 bottom
R23  18.22,5.29 0 bottom
R28  4.47,7.01 0 bottom
R29  4.5,5.91 0 bottom
S1  16.71,10.41 270 top
S2  7.78,10.41 270 top
S3  16.71,28.83 90 top
SDPC  2.6,18.68 270 bottom
U1  11.43,49.91 90 top
U3  6.57,25.63 270 top
U4  12.6,27.94 90 top
U5  6.14,30.65 90 top
U6  16.13,16.89 0 top
U$1  [#17#11]  3.16,36.83 0 top
U$2  [BOOT0]  9.78,10.52 90 top
U$3  [#MEAS#1714141838]  6.34,21.49 0 bottom
U$4  [IO180]  14.66,35.5 0 top
U$5  [NORA#W3060]  11.39,39.76 0 top
U$6  [##RST##23061714141845]  21.58,11.72 90 bottom
U$7  [USER0]  16.76,25.78 0 top
U$8  [SFE_LOGO_FLAME_.2]  7.22,35.74 0 top
U$9  [IO20]  16.86,31.93 0 top
U$10  [#GND#ON#3061714141842]  2.56,14.06 90 bottom
U$11  [#SDPC#0]  1.05,18.51 90 bottom
U$12  [#A0#1]  19.44,24.12 0 bottom
U$13  [#SDA#11#28]  5,52.05 0 bottom
U$14  [#17#28]  3.15,36.83 0 bottom
U$15  [#0#4]  20.06,26.64 0 bottom
U$16  [#1#4]  20.22,29.22 0 bottom
U$17  [#SCL#12#28]  5.02,49.57 0 bottom
U$18  [#18#28]  3.11,34.27 0 bottom
U$19  [SFE_LOGO_FLAME_.1]  12.48,50.73 0 bottom
U$20  [#LD#29]  3.38,31.72 0 top
U$21  [RGB_IO140]  15.66,37.45 0 top
U$22  [#17#11]  2.61,21.47 90 bottom
U$23  [PWR0]  14.73,34.25 0 top
U$24  [#CUR#0]  10.4,26.8 90 bottom
U$25  [THING_PLUS1714141839]  11.41,56.66 0 bottom
U$26  [#VB26]  3.08,24.09 0 bottom
U$28  [NORA#W3061714141840]  11.43,54.95 0 bottom
U$30  [#13#13]  3.22,47.03 0 bottom
U$31  [#14#14]  3.17,44.48 0 bottom
U$32  [#15#15]  3.13,41.87 0 bottom
U$33  [#16#16]  3.14,39.37 0 bottom
U$35  [#18#18]  3.11,34.27 0 top
U$36  [#11#91420]  3.03,52.06 0 top
U$37  [#12#91420]  3.21,49.55 0 top
U$38  [#13#91420]  3.19,47.02 0 top
U$39  [#14#91420]  3.14,44.48 0 top
U$40  [#15#91420]  3.12,41.89 0 top
U$41  [#VUSB#0]  1.5,29.21 0 bottom
U$42  [#JP3#23061714141846]  12.53,35.87 90 bottom
U$43  [#EN#0]  1.5,26.67 0 bottom
U$44  [#16#91420]  3.15,39.37 0 top
U$45  [#3V3#0]  21.19,16.52 0 bottom
U$46  [#NC#2]  19.53,19.03 0 bottom
U$47  [#A0#18]  19.76,24.11 0 top
U$48  [#8#91421]  20.03,46.95 0 top
U$49  [#7#8]  20.06,44.41 0 top
U$50  [#6#8]  20.04,41.88 0 top
U$51  [#5#8]  20.07,39.33 0 top
U$52  [#4#8]  20.04,36.79 0 top
U$53  [#3#8]  20.03,34.29 0 top
U$54  [#2#8]  20.03,31.74 0 top
U$55  [#1#8]  20.22,29.22 0 top
U$56  [#0#8]  20.05,26.64 0 top
U$57  [#3V#23]  19.8,16.53 0 top
U$58  [#JP2#0]  5.79,36.49 90 bottom
U$59  [ORDERING_INSTRUCTIONS]  not placed on the board
U$60  [#SWD#501]  15.9,18.79 90 bottom
U$61  [#100#23061714141846]  6.53,27.6 0 bottom
U$62  [THING_PLUS_0]  11.57,41.13 0 top
U$63  [#SHLD#9]  9.94,2.75 0 bottom
U$64  [#GND#10]  18.91,21.55 0 bottom
U$65  [#JP1#0]  8.06,38.45 90 bottom
U$66  [#PWR#14]  10.39,35.41 90 bottom
U$67  [#CHG#13]  13.4,29.05 90 bottom
U$68  [##RESET##19]  21.62,10.53 90 top
U$69  [#NC#21]  19.69,19.14 0 top
U$70  [#9#10]  20.08,49.54 0 top
U$71  [#LED_DO#0]  5.02,31.81 0 bottom
U$72  [#I2C#3]  3,7.68 90 bottom
U$73  [#500#23061714141846]  6.42,25.75 0 bottom
U$74  [#10#11]  19.74,52.11 0 top
U$75  [#G#22]  20.06,21.6 0 top
U$76  [#VU#23]  3.15,29.24 0 top
U$77  [#VB26]  3.16,24.03 0 top
U$78  [CHG0]  14.57,32.99 0 top
U$79  [RESET0]  18.7,10.43 90 top
U$80  [#EN#27]  3.14,26.66 0 top
U$81  [#2#28]  20.03,31.73 0 bottom
U$82  [#3#28]  20.03,34.29 0 bottom
U$83  [#4#CS#28]  18.65,36.79 0 bottom
U$84  [#5#SCK#28]  18.22,39.32 0 bottom
U$85  [#6#PICO#28]  17.85,41.88 0 bottom
U$86  [#7#POCI#28]  17.89,44.42 0 bottom
U$87  [#9#TX1#A2#28]  16.74,49.53 0 bottom
U$88  [#8#RX1#A1#28]  16.92,46.94 0 bottom
U$91  [#10#28]  19.74,52.11 0 bottom
USBSHLD  6.55,2.97 180 bottom

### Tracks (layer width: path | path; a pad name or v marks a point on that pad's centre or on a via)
3.3V  (via drill 0.2)
  Top 0.178: 9.95,42.51 9.94,42.52 v10.04,42.63 | C1.1 | v3.95,9.9 v3.95,9.89 3.09,9.89 2.42,9.22 v2.42,7.68
  Top 0.254: 9.23,42.51 C4.1
  Top 0.508: U1.A7 U1.A8 | U1.A7 U1.B7 | C4.1 9.95,42.51 | U1.A7 9.23,42.51 | C1.1 8.72,29.08 | v9.21,30.07 9.21,29.56 8.72,29.08 | C1.1 C10.1 8.73,26.68 8.62,26.58 U3.5 | J3.2 v3.95,9.9 | v7.82,20 v7.82,19.99 v8.37,19.99 v8.38,19.98 11.66,19.98 11.7,20.02 11.7,19.58 v11.69,19.57 | v7.82,29.09 8.32,29.09 v8.33,29.08 8.72,29.08
  Bottom 0.178: v9.53,34.4 10.43,34.4 10.86,33.98 LED.1 | I2C.2 1.45,7.68 v2.42,7.68 | J6.1 13.75,21.95 14.56,22.76 v14.56,22.81 | R20.1 19.84,6.86 Q4.2 | JP3.1 11.66,38.3 11.4,38.55 v11.4,38.9
  Bottom 0.508: v20.81,7.48 20.51,7.77 Q4.2 | Q3.2 R19.1 7.6,19.78 v7.82,20
  other vias: 10.69,42.61 10.69,41.91 10.05,41.9 9.2,30.58 9.71,30.57 9.71,30.06 11.66,20.03
  pour Route15 (isolate 0.305, rank 2): 0,58.37 7.14,58.37 7.14,54.36 15.7,54.36 15.7,58.37 22.86,58.37 22.86,0 0,0
  pour Top (isolate 0.305): 10.99,42.92 9.7,42.92 9.7,41.63 10.99,41.63
  pour Top (isolate 0.203): 9.95,29.83 8.98,29.83 8.98,30.85 9.95,30.85
!RESET!  (via drill 0.2)
  Top 0.178: S1.1 15.91,10.16 | 15.91,10.16 S1.2 | v20.19,22.95 20.17,22.95 19.77,23.36 19.77,24.51 18.94,25.33 16.11,25.33 15.16,24.38 v15.16,23.36 | v15.84,21.97 Q2.3 | U1.J3 14.18,52.66 17.62,52.66 19.09,51.19 19.09,46.27 18.3,45.49 18.3,43.11 17.32,42.13 17.32,37.76 v15.8,36.24 | J1.28 21.59,9.75 20.98,9.14 C11.1 18.83,9.14 17.8,10.16 15.91,10.16
  Bottom 0.178: v20.19,22.95 20.11,22.86 20.11,16.31 21.11,15.31 21.34,15.31 21.59,15.06 J1.28 | v15.16,23.36 15.16,22.64 v15.84,21.97 | v15.8,36.24 15.8,33.28 16.48,32.6 16.48,24.68 v15.16,23.36 | J6.10 11.77,16.24 12.09,16.56 12.09,17.11 11.68,17.52 11.68,18.73 12.31,19.36 12.31,21.86 13.81,23.36 v15.16,23.36
CC1
  Top 0.178: R12.2 10.18,13.57 J5.A5
CC2
  Top 0.178: J5.B5 13.18,6.91 14.34,8.07 R11.2
CHG  (via drill 0.2)
  Top 0.178: U4.1 14.9,26.99 v14.92,26.97
  Bottom 0.178: CHG.2 12.84,29.05 v14.92,26.98 v14.92,26.97
DTR
  Top 0.178: Q2.1 16.05,23.27 15.91,23.4 | 15.91,23.4 15.81,23.51 15.81,24.48 16.06,24.73 R17.1 | 15.91,23.4 14.89,22.38 14.89,20.16 15.38,19.68 U6.23
EN
  Top 0.178: U3.3 3.26,24.68 J1.11 2.48,27.88 R8.2
GND  (via drill 0.2)
  Top 0.178: 14.73,45.5 U1.B2 | 8.12,45.51 U1.B8 | v7.57,44.96 7.57,44.95 | v15.27,44.96 v15.28,44.96 | U6.2 14.95,17.64 | U6.PAD v16.13,17.52 v16.14,17.53 | U5.4 7.88,31.4 | 7.88,31.4 7.95,31.4 C15.2 | U5.1 7.13,29.58 7.05,29.5 6.15,29.5 6.1,29.55 | U5.6 4.7,30.9 4.58,31.02 4.58,31.73 4.59,31.74 | 7.88,31.4 7.84,31.44 7.84,32.4 | v14.53,25.18 15.12,25.77 15.12,26.04 15.86,26.78 S3.4 | v15.27,57.31 | v15.27,57.31 15.12,57.31 v15.27,57.31 | U1.M2 | U1.M2 v15.27,57.31 | U1.M8 v7.57,57.31
  Top 0.203: C10.2 7.68,27.39 7.21,27.39 6.97,27.15 v6.64,27.15 | C1.2 7.22,28.4 6.99,28.63
  Top 0.406: v15.27,44.96 14.73,45.5 v14.16,46.06 | v7.57,44.96 8.12,45.51 v8.66,46.06 | 7.57,44.95 U1.A9 | v15.28,44.96 U1.A1
  Bottom 0.178: v14.67,7.63 14.09,7.63 J4.6
  other vias: 7,55.04 7.01,56.55 6.34,57.32 15.84,55.04 15.83,56.56 16.55,57.31 8.67,54.31 9.77,54.31 13.07,54.31 14.17,54.31 11.97,49.36 11.42,49.91 10.87,49.36 11.42,48.81 11.97,48.26 12.52,48.81 12.52,49.91 10.32,49.91 10.32,48.81 10.87,48.26 7.02,43.86 6.47,44.41 15.82,43.86 16.37,44.41 11.97,54.31 10.87,54.31 16.53,55.82 6.35,55.81 12.52,51.56 12.52,52.66 10.32,51.56 10.32,52.66 12.52,53.76 10.32,53.76 11.43,7.8 15.06,27.94 6.8,14.45 4.06,25.46 11.52,24.02 12.17,17.71 16.13,16.85 15.45,16.9 16.82,16.87 16.11,16.16 9.64,36.23 8.16,13.75 14.54,13.08 20.7,12.14 17.78,0.56 5.13,0.57 0.54,5.18 0.54,10.15 0.54,15.64 0.54,19.94 11.57,16.82 5.96,15.75 8.34,17.83 5.21,56.39 0.76,53.85 17.65,56.39 21.72,53.59 15.04,32.03 15.02,28.9 8.95,22.14 4.51,35.2 13.26,36.15 13.63,34.37 15.85,38.06 3.81,10.92 5.08,11.68 7.62,6.99 5.71,4.83 3.25,53.51 4.55,54.35 5.69,29.33 3.07,7.18 15.38,20.87 17.68,22.43 16.5,23.93 17.81,40.97 19.7,45.38 10.23,31.35 8.88,33.35 5.4,55.44 20.55,40.78 19.36,44.03 17.9,51.37 16.69,53.19 17.51,45.61 12.23,14.26 18.62,12.51 7.2,38.64 7.22,41.62 4.99,40.24 5.66,51.57 0.56,35.57 0.55,38.12 22.31,33.04 22.29,25.41 18.28,15.01 4.07,25.93 6.16,32.05 16.47,41.28 15.21,41.36 13.98,39.98 5,39 4.95,36.91 21.04,25.42 19.63,42.93 17.93,31.82 3.61,31.04 1.83,30.48 6.33,48.72 3.44,16.65 4.19,20.91 7.35,20.72 14.25,26.32 3.54,27.21 1.99,16.94 17.91,19.6 11.54,21.61 17.49,48.1 22.29,48.24
  pour Route2 (isolate 0.305): 0,57.53 7.16,57.5 8.33,57.5 8.33,57.11 7.17,57.11 7.16,54.36 15.67,54.36 15.69,57.11 14.53,57.11 14.53,57.51 22.86,57.51 22.86,0 0,0
  pour Top (isolate 0.178, rank 4): 0,0 0,58.42 22.86,58.42 22.86,0
  pour Bottom (isolate 0.152, rank 2): 0,0 22.86,0 22.86,58.42 0,58.42
N$1
  Top 0.178: U6.9 15.88,13.97 16.23,13.61 17.71,13.61 18.6,14.51 R1.2
N$2
  Top 0.178: R4.2 8.84,35 9.39,35.56 D3.A
N$3
  Top 0.178: R17.2 18.89,24.73 19.32,24.31 19.32,22.84 19.1,22.62 Q2.5
N$4
  Top 0.178: U6.8 15.38,13.83 15.98,13.23 19.12,13.23 R5.1 19.85,12.49 R9.2
N$5
  Top 0.178: R18.2 16.08,20.87 15.34,21.6 15.34,22.18 15.78,22.62 Q2.2
N$6  (via drill 0.2)
  Top 0.178: D1.C 13.67,33.02 v13.69,33
  Bottom 0.178: v13.69,33 13.69,32.64 13.88,32.44 CHG.1
N$7
  Top 0.178: R10.2 12.94,21.5 Q1.1
N$8
  Top 0.178: S2.3 S2.4 8.58,13.5 8.68,13.6 R15.2
N$9  (via drill 0.2)
  Top 0.178: U4.5 v10.27,26.99 v10.26,27
  Bottom 0.178: v10.26,27 10.02,26.75 CUR.2
N$10  (via drill 0.2)
  Top 0.178: D5.DI 12.74,36.95 12.85,36.84 v13.24,36.84
  Bottom 0.178: v13.24,36.84 9.39,36.84 9.01,36.47 JP1.2
N$11  (via drill 0.2)
  Top 0.178: v8.99,24.19 9,24.21 R13.1
  Bottom 0.178: CUR.1 8.08,27.79 6.93,26.64 6.93,25.11 7.33,24.72 8.46,24.72 v8.99,24.19
N$12  (via drill 0.2)
  Top 0.178: v8.69,32.67 8.39,32.37 R2.1 | v8.69,32.67
  Bottom 0.178: LED.2 8.74,32.72 v8.69,32.67
N$13  (via drill 0.2)
  Top 0.178: v7.43,25.36 7.53,25.47 R6.2
  Bottom 0.178: v7.43,25.36 7.77,25.7 CUR.3
N$14
  Top 0.178: D4.A 9.39,33.13 R2.2
N$15
  Top 0.203: D6.6 10.93,10.48 11.24,10.79 11.24,15.19 13.2,17.14 U6.3
N$16
  Top 0.203: D6.1 10.93,7.51 11.18,7.26 J5.A6 11.18,4.57 11.44,4.3 11.96,4.3 12.18,4.52 J5.B6
N$17
  Top 0.178: D1.A 10.55,32.13 R3.2
N$18
  Top 0.178: D6.4
  Top 0.203: D6.4 11.93,10.46 11.6,10.79 11.6,15.04 13.21,16.64 U6.4
N$19  (via drill 0.2)
  Top 0.178: v10.68,4.88 v10.68,4.87 | J5.A7
  Top 0.203: J5.A7 11.68,7.29 11.93,7.54 D6.3 | J5.B7 v10.68,4.88 | J5.A7 v11.68,4.87
  Bottom 0.178: v10.68,4.87 v10.69,4.87
  Bottom 0.203: v10.69,4.87 v11.68,4.87
N$20
  Bottom 0.178: R28.2 2.32,8.66 I2C.3
N$21
  Bottom 0.178: R29.2 3.21,5.91 2.55,6.58 I2C.1
N$22  (via drill 0.2)
  Top 0.178: v7.15,33.78 7.46,34.08 R4.1
  Bottom 0.178: JP2.2 6.54,34.39 v7.15,33.78
N$23
  Top 0.178: 11,20.87 Q1.2
  Top 0.508: 11,20.87 D2.C 8.24,20.87 7.64,21.46 MEAS.3
  Bottom 0.178: MEAS.1 MEAS.3
N$24
  Bottom 0.178: Q3.1 R14.2
N$25  (via drill 0.2)
  Top 0.178: C5.1 13.05,8.33 12.76,8.04 v12.44,8.04
  Route15 0.178: v12.44,8.04 11.62,8.86 10.8,8.86 6.05,13.61 v4.75,13.61
  Bottom 0.178: J4.4 11.89,7.48 v12.44,8.04 | R16.1 4.45,13.31 v4.75,13.61
  Bottom 0.508: v4.75,13.61 4.86,13.72 4.86,16.07 Q3.3
N$26
  Bottom 0.178: SDPC.2 3.46,18.68 3.61,18.54 3.61,17.86 3.89,17.58 5.38,17.58 | 5.38,17.58 7.55,17.58 R19.2 | R14.1 5.38,17.59 5.38,17.58
N$27
  Bottom 0.178: Q5.3 18.76,6.28 19.4,5.64 20.59,5.64 | R21.2 20.59,5.64 | R20.2 20.59,5.64
N$28  (via drill 0.2)
  Top 0.178: v13.22,39.38 13.4,39.19 C8.1 12.71,38.45 D5.VCC
  Bottom 0.178: JP3.2 v13.22,39.37 v13.22,39.38
N$29  (via drill 0.2)
  Top 0.178: U6.5 13.46,16.14 13.21,15.89 | 13.67,13.79 13.67,14.05 12.93,14.79 12.93,15.6 13.21,15.89 | 13.67,13.79 v13.67,13.07 | U6.6 13.46,15.64 13.21,15.89 | U6.7 14.88,14.01 14.66,13.79 13.67,13.79 | R1.1 20.39,15.51 20.55,15.35 v20.55,14.91
  Top 0.254: C3.1 13.14,11.54 13.7,12.09 | v13.67,13.07 13.67,12.12 13.7,12.09 | C2.1 13.73,12.06 13.7,12.09
  Route15 0.254: v20.92,8.59 18.15,8.59 v13.67,13.07
  Bottom 0.178: v20.92,8.59 20.92,9.75 Q4.3 21.49,10.56 21.49,12.29 20.32,13.45 20.32,14.67 v20.55,14.91
N$30
  Bottom 0.178: Q4.1 21.77,7.75 R21.1
N$31
  Bottom 0.178: Q5.1 17.72,6 R23.2
N$32
  Bottom 0.178: SDPC.3 2.6,16.69 3.6,15.69 R22.1
PA7/UART-LOG-TXD  (via drill 0.2)
  Top 0.178: v17.45,23.25 17.47,23.27 Q2.6 | v4.47,12.56 4.57,12.46 S2.1 S2.2 | U6.20 16.88,19.71 v16.31,20.27 | J1.22 20.35,30.45 20.35,31.23 17.92,33.67 v17.47,33.67 | U1.A5 11.43,43.83 15.7,39.56 v15.93,39.56
  Bottom 0.178: v4.47,12.56 5.4,13.48 5.4,14.49 6.51,15.61 16.34,15.61 17.49,16.75 17.49,19.1 v16.31,20.27 17.18,21.14 17.18,22.97 v17.45,23.25 17.45,33.65 v17.47,33.67 16.9,34.23 16.9,38.59 v15.93,39.56
PA8/UART-LOG-RXD  (via drill 0.2)
  Top 0.178: U6.21 16.38,19.6 16.21,19.77 15.8,19.77 15.64,19.93 v15.64,20.27 | J1.23 21.59,26.7 19.91,28.38 19.91,30.76 17.71,32.96 17.28,32.96 v16.88,33.35 | v15.94,38.79 15.93,38.79 10.33,44.39 U1.A6
  Bottom 0.178: v15.64,20.27 15.64,20.42 16.71,21.48 16.71,23.39 17.1,23.79 17.1,33.13 v16.88,33.35 16.5,33.74 16.5,38.24 v15.94,38.79
PA12  (via drill 0.2)
  Top 0.178: U1.J9 5.51,53.21 2.81,50.51 2.81,45.38 1.89,44.45 J1.4 3.3,42.42 v3.34,42.42
  Bottom 0.178: v3.34,42.42 v3.35,42.41 3.35,37.17 4.15,36.37 6.2,36.37 7.15,35.42 JP1.1
PA13
  Top 0.178: U1.J8 7.58,53.76 5.61,53.76 2.47,50.62 2.47,48.19 J1.3
PA14
  Top 0.178: U1.H9 5.42,52.11 3.48,50.17 3.48,43.62 4.19,42.91 4.19,41.97 3.77,41.54 3.44,41.54 J1.6
PA15
  Top 0.178: U1.H8 7.58,52.66 5.42,52.66 3.15,50.38 3.15,43.42 3.85,42.71 3.85,42.18 3.58,41.91 J1.5
PA25/SCL  (via drill 0.2)
  Top 0.178: v3.88,7.89 v3.88,7.9 J3.4 | U5.7 3.7,30.4 3.63,30.48 v2.54,30.48 | J1.2 1.27,50.59 1.48,50.8 1.92,50.8 v2.65,51.54 | v14.18,48.26 14.18,47.16 U1.C2
  Bottom 0.178: J1.2 2.54,48.26 v2.54,30.48 2.54,23.55 1.04,22.05 1.04,10.73 v3.88,7.89 4.65,7.89 4.97,7.57 R28.1 | v14.18,48.26 13.49,47.57 8.4,47.57 7.74,48.22 4.06,48.22 3.25,49.03 3.25,50.94 v2.65,51.54
PA26/SDA  (via drill 0.2, 0.2 pad 0.25)
  Top 0.178: v3.87,8.89 J3.3 | U5.8 3.12,29.9 3.11,29.91 v3.09,29.91 | U1.C1 v15.29,47.15
  Bottom 0.178: J1.1 1.27,51.82 2.85,50.23 2.85,47.78 | 2.85,47.78 2.85,32.95 3.09,32.71 v3.09,29.91 3.09,23.34 1.52,21.77 1.52,11.24 v3.87,8.89 4.81,8.89 5.91,7.79 5.91,6.14 5.69,5.91 R29.1 | v15.29,47.15 8.29,47.15 7.67,47.78 2.85,47.78
PA27/SWD_DATA  (via drill 0.2)
  Top 0.178: U1.H2 15.28,51.56 16.84,51.56 v16.86,51.54 v16.86,51.53 v16.86,48.09 | v15.83,40.95 15.83,43.02 v16.59,43.78
  Bottom 0.178: v16.86,51.54 17.39,52.07 J1.13 | J6.2 10.82,21.32 10.96,21.45 10.96,22.3 15.56,26.91 15.56,32.2 14.55,33.21 14.55,39.67 v15.83,40.95 | v16.59,43.78 16.85,44.04 v16.85,48.09 v16.86,48.09
PA28  (via drill 0.2)
  Top 0.178: U1.B3 13.63,45.49 13.08,44.93 13.08,42.77 15.55,40.3 v15.93,40.3 | v17.47,35.53 18.09,35.53 18.42,35.2 20.68,35.2 J1.20
  Bottom 0.178: v15.93,40.3 17.47,38.75 v17.47,35.53
PA30
  Top 0.178: U1.B1 16.42,45.51 17.62,44.31 17.62,42.98 16.97,42.33 16.97,38.12 15.26,36.4 15.26,35.17 15.96,34.46 | J1.21 18.88,34.46 15.96,34.46 | S3.1 S3.2 16.02,32.37 16.02,34.4 15.96,34.46
PB1/LP_UART_TXD/A2  (via drill 0.2)
  Top 0.178: v8.67,48.25 U1.D8
  Bottom 0.178: J1.14 21.59,49.96 20.82,50.72 15.48,50.72 14.05,52.15 9.52,52.15 7.73,50.37 7.73,49.1 8.58,48.25 v8.67,48.25
PB2/LP_UART_RXD/A1  (via drill 0.2)
  Top 0.178: U1.E8 v8.67,49.35
  Bottom 0.178: J1.15 19.77,46.99 18.41,48.34 18.41,49.45 17.84,50.03 14.37,50.03 13.51,50.89 10.21,50.89 v8.67,49.35
PB3/SWD_CLK/A0  (via drill 0.2)
  Top 0.178: U1.J2 15.28,53.76 18.57,53.76 20.27,52.06 v20.27,42.87 | J1.24 19.82,25.91 16.08,25.91 14.41,24.24 v14.41,24.22
  Bottom 0.178: v20.27,42.87 20.27,42.42 20.08,42.23 20.08,25.64 J1.24 | v14.41,24.22 13.92,24.22 12,22.29 12,21.25 10.79,20.05 J6.4
PB18/SPI0_PICO  (via drill 0.2)
  Top 0.178: J1.17 20.05,41.91 v18.64,41.91 | U1.G9 6.99,50.97 6.43,50.97 5.14,49.68 5.14,43.63 5.71,43.05 v5.71,40.02
  Bottom 0.178: J4.3 10.79,7.61 10.04,8.36 7.86,8.36 7.64,8.58 7.64,14.12 8.29,14.77 16.97,14.77 18.9,16.7 18.9,39.49 18.65,39.74 18.65,41.9 v18.64,41.91 18.3,42.25 14.7,42.25 12.27,39.82 5.91,39.82 v5.71,40.02
PB19/SPI0_POCI  (via drill 0.2)
  Top 0.178: U1.G8 7.58,51.56 6.47,51.56 4.8,49.9 4.8,43.52 5.23,43.09 v5.23,40.95
  Bottom 0.178: J4.7 15.19,7.6 15.33,7.74 18.42,7.74 18.83,8.15 18.83,11.26 19.69,12.12 19.69,42.2 18.93,42.96 | J1.16 20.64,43.49 19.52,43.49 18.99,42.96 18.93,42.96 | v5.23,40.95 12.4,40.95 14.42,42.96 18.93,42.96
PB20/SPI0_CLK  (via drill 0.2)
  Top 0.178: J1.18 20.77,40.19 v19.2,40.19 | v6.72,40.36 6.72,42.95 5.81,43.86 5.81,49.15 6.58,49.91 U1.F9
  Bottom 0.178: J4.5 12.99,7.13 13.99,8.13 18.16,8.13 18.41,8.38 18.41,11.47 19.27,12.32 19.27,39.64 19.2,39.71 v19.2,40.19 19.2,42.23 18.82,42.61 14.57,42.61 12.34,40.38 6.74,40.38 v6.72,40.36
PB21/SPI0_CS  (via drill 0.2)
  Top 0.178: J1.19 21.57,36.81 v18.41,36.81 | U1.F8 7.58,50.46 6.47,50.46 5.49,49.48 5.49,43.72 6.2,43.02 v6.2,39.34
  Bottom 0.178: J4.2 9.69,7.75 9.42,8.02 7.11,8.02 5.89,9.25 5.89,12.53 | 5.89,12.53 5.89,14.21 6.76,15.09 16.84,15.09 18.41,16.66 18.41,36.27 18.41,36.26 v18.41,36.81 18.41,39.46 18.33,39.55 18.33,41.44 17.86,41.9 14.87,41.9 12.38,39.41 6.26,39.41 v6.2,39.34 | R16.2 4.08,11.9 4.61,11.9 5.24,12.53 5.89,12.53
PB22  (via drill 0.2)
  Top 0.178: 3.75,34.29 v4.75,33.29 | J1.8 3.75,34.29 | U1.E9 7.58,48.26 v7.58,47.16 | v4.24,37.39 4.48,37.15 4.48,35.97 3.75,35.25 3.75,34.29
  Bottom 0.178: v7.58,47.16 5.09,47.16 3.82,45.89 3.82,37.8 v4.24,37.39 | JP2.1 5.71,33.29 v4.75,33.29
PB23/SDPC  (via drill 0.2)
  Top 0.178: v7.6,46.08 | U1.C8 v7.6,46.08 | v4.34,38.93 3.37,38.93 J1.7 2.92,36.83 v3.41,36.34
  Bottom 0.178: v7.6,46.08 4.52,46.08 4.19,45.76 4.19,39.56 4.34,39.42 v4.34,38.93 | v3.41,36.34 3.41,33.12 4.1,32.44 4.1,27.07 3.58,26.55 3.58,22.48 2.6,21.5 SDPC.1
RTS
  Top 0.178: Q2.4 19.06,21.97 19.3,21.73 19.3,21.12 19.04,20.87 R18.1 17.95,20.35 17.38,19.78 U6.19
USB_SHLD  (via drill 0.2)
  other vias: 8.52,0.93
  pour Top (isolate 0.254, rank 2): 16.15,5.31 6.73,5.31 6.73,0.76 16.15,0.76
  pour Bottom (isolate 0.254): 6.73,0.76 16.15,0.76 16.15,5.84 6.73,5.84
V_BATT  (via drill 0.2)
  Top 0.178: 11.95,18.78 Q1.3 | v7.15,29.07 7.15,29.13 7.61,29.59 7.83,29.59 C15.1 7.96,30.39 7.77,30.39 | U5.2 7.77,30.39 | U5.3 7.66,30.9 7.67,30.91 7.77,30.8 7.77,30.39
  Top 0.508: J1.12 2.06,24.13 5.38,20.8 6.07,20.8 7.18,19.69 J2.2 11.95,18.78 | Q1.3 12.61,18.74 13.74,19.86 13.74,21.75 13.25,22.24 13.25,26.05 12.88,26.42 12.88,28.61 13.16,28.89 U4.3 14.08,28.89 14.13,28.94 14.13,30.17 C6.1
  Route15 0.178: J1.12 3.41,24.13 4.85,25.57 4.85,27.55 6.37,29.07 v7.15,29.07
V_USB  (via drill 0.2)
  Top 0.178: D6.5 v11.43,10.11 | R5.2 19.48,13.87 v18.74,13.87 | v10.21,22.96 10.47,23.22 | R3.1 11.93,31.26 11.79,31.12 11.14,31.12 10.93,30.91 C19.1
  Top 0.508: D2.A 10,23.17 v10.21,22.96 | 10.47,23.22 R7.2 11.19,22.27 R10.1 | v9.58,28.88 v10.13,28.88 v10.14,28.89 U4.4 10.93,28.89 C19.1
  Route15 0.178: v18.74,13.87 16.17,13.87 14.56,15.47 10.21,15.47 | 10.21,15.47 | v13.11,3.53 14.63,3.53 14.75,3.41 v17.16,3.41 | v17.16,3.41
  Route15 0.508: J1.10 3.94,29.21 5.08,30.35 7.96,30.35 9.43,28.88 v9.58,28.88 9.58,25.6 10.21,24.97 v10.21,22.96 v10.21,22.42 10.21,15.47 10.21,11.33 v11.43,10.11 12.55,10.11 13.83,8.83 13.83,6.41 13.12,5.71 v13.12,4.08
  Bottom 0.178: R23.1 17.89,4.46 17.62,4.46 17.16,4 v17.16,3.41
  other vias: 12.54,4.1 12.54,3.52
  pour Top (isolate 0.178, no thermals): 13.24,3.3 9.53,3.3 8.78,4.05 8.78,6.16 14.08,6.16 14.08,4.15
  pour Route15 (isolate 0.305): 13.24,4.2 12.41,4.2 12.41,3.38 13.24,3.38
  pour Route15 (isolate 0.305): 9.39,29.04 10.32,29.04 10.32,28.73 9.39,28.73
  pour Top (isolate 0.305): 11.43,23.43 9.68,23.43 9.68,21.84 11.43,21.84
VIN
  Top 0.178: R8.1 4,27.84 4,26.98 4.41,26.58 U3.1
  Top 0.508: U3.1 5.66,26.58 | 5.66,26.58 5.79,26.58 6.3,26.07 6.3,24.21 MEAS.4 | C7.1 5.65,26.59 5.66,26.58
  Bottom 0.178: MEAS.2 MEAS.4
WS2812-DO
  Top 0.178: J1.9 1.27,31.96 2.61,33.29 4.04,33.29 4.55,32.78 5.64,32.78 6.21,33.34 6.21,35.78 6.8,36.38 8.47,38.05 D5.DO

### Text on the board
Top: 1
Route2: 2
Route15: 3
Bottom: v10 | 4
tPlace: + | -
Measures: Measure Units: INCHES
Reference: 11 | 10 | 12 | 9 | 13 | 8 | 14 | 7 | 15 | 6 | 16 | 5 | 17 | 4 | 18 | 3 | LD | 2 | VU | 1 | EN | 0 | vbat | A0 | G | 3.3V | RESET
tDocu: Soldermask: Red / Thickness: 1.6mm / Four Layer Design / 1oz copper outer / 0.5oz copper inner / Finish: HASL / Stackup: JLC7628 / Material: TG155 | Pete Lewis | Based on designs by: M. Hord, A. Wende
